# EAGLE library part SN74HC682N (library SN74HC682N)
Magnitude Comparator 8-Bit 20-Pin PDIP Source: Datasheet
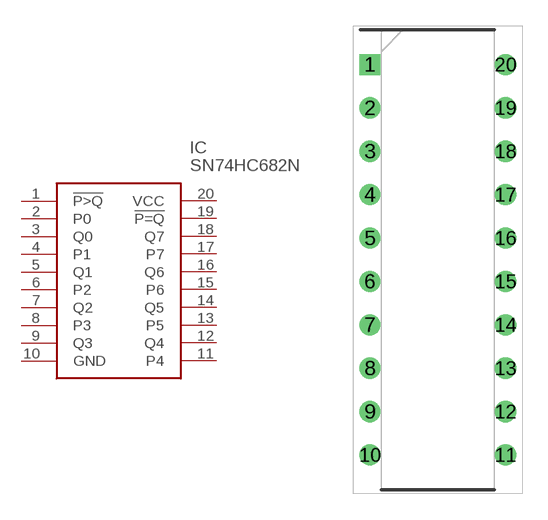
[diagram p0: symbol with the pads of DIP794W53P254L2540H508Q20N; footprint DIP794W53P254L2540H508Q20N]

Designator prefix IC

## SN74HC682N (Description: Magnitude Comparator 8-Bit 20-Pin PDIP; Height: 5.08mm; Manufacturer_Name: Texas Instruments; Manufacturer_Part_Number: SN74HC682N; Mouser_Part_Number: 595-SN74HC682N; Mouser_Price-Stock: https://www.mouser.co.uk/ProductDetail/Texas-Instruments/SN74HC682N?qs=JD1fk4stihZ5fZizX5ugBQ%3D%3D)  [DIP794W53P254L2540H508Q20N]
1  !P>Q
2  P0
3  Q0
4  P1
5  Q1
6  P2
7  Q2
8  P3
9  Q3
10  GND
11  P4
12  Q4
13  P5
14  Q5
15  P6
16  Q6
17  P7
18  Q7
19  !P=Q
20  VCC

## Footprint DIP794W53P254L2540H508Q20N (pad centres in mm)
N (R-PDIP-T)
drill 0.73 pad 1.13 square: 1 -3.97,11.43
drill 0.73 pad 1.13: 2 -3.97,8.89; 3 -3.97,6.35; 4 -3.97,3.81; 5 -3.97,1.27; 6 -3.97,-1.27; 7 -3.97,-3.81; 8 -3.97,-6.35; 9 -3.97,-8.89; 10 -3.97,-11.43; 11 3.97,-11.43; 12 3.97,-8.89; 13 3.97,-6.35; 14 3.97,-3.81; 15 3.97,-1.27; 16 3.97,1.27; 17 3.97,3.81; 18 3.97,6.35; 19 3.97,8.89; 20 3.97,11.43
